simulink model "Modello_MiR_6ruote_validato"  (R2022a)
settings: Solver=VariableStepAuto  StartTime=0.0  StopTime=time_s(end,1)  RelTol=1e-3
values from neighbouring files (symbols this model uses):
  a = 0.250    (= 0.25)    [Modello_MiR_6ruote_validato_script.m]    (also in Modello_MiR_2ruote_script.m; Modello_MiR_6ruote_script.m; Modello_MiR_UR_script.m)
  a1 = 0.18265    [Modello_MiR_6ruote_validato_script.m]    (also in Modello_MiR_2ruote_script.m = deg2rad(5); Modello_MiR_6ruote_script.m = deg2rad(5); Modello_MiR_UR_script.m; UR_DHtable_e.m = 0)
  a2 = 0.40857    [Modello_MiR_6ruote_validato_script.m]    (also in Modello_MiR_2ruote_script.m = deg2rad(25); Modello_MiR_6ruote_script.m = deg2rad(25); Modello_MiR_UR_script.m; UR_DHtable_e.m = 612)
  Att_C1 = 0.01    [Modello_MiR_6ruote_validato_script.m]    (also in Modello_MiR_UR_script.m)
  Att_C2 = 0.01    [Modello_MiR_6ruote_validato_script.m]    (also in Modello_MiR_UR_script.m)
  Att_C5 = 0.01    [Modello_MiR_6ruote_validato_script.m]    (also in Modello_MiR_UR_script.m)
  Att_C6 = 0.01    [Modello_MiR_6ruote_validato_script.m]    (also in Modello_MiR_UR_script.m)
  b = 0.1875    [Modello_MiR_6ruote_validato_script.m]    (also in Modello_MiR_2ruote_script.m; Modello_MiR_6ruote_script.m; Modello_MiR_UR_script.m)
  b_caster = 0.07    [Modello_MiR_6ruote_validato_script.m]    (also in Modello_MiR_2ruote_script.m; Modello_MiR_6ruote_script.m; Modello_MiR_UR_script.m)
  bd = 0.205    [Modello_MiR_6ruote_validato_script.m]    (also in Modello_MiR_2ruote_script.m; Modello_MiR_6ruote_script.m; Modello_MiR_UR_script.m)
  F23fun = @(u) (mv*9.801/4)-(mv*h*u(5)+(mv*9.801/4)*(2*a-b_caster*(cos(u(1))+cos(u(2)))))/(4*a-b_caster*(cos(u(1))+cos(u(2)))+b_caster*(cos(u(3))+cos(u(4))))    [Modello_MiR_6ruote_validato_script.m]    (also in Modello_MiR_6ruote_script.m = @(u) (mv*9.801/4)-u(7))
  F43fun = @(u) (1/(2*bd))*(mv*u(6)*h+((mv*h*u(5)+(mv*9.801/4)*(2*a-b_caster*(cos(u(1))+cos(u(2)))))/(4*a-b_caster*(cos(u(1))+cos(u(2)))+b_caster*(cos(u(3))+cos(u(4)))))*(2*bd-b_caster*(sin(u(3))+sin(u(4))))+((mv*9.801/4)-(mv*h*u(5)+(mv*9.801/4)*(2*a-b_caster*(cos(u(1))+cos(u(2)))))/(4*a-b_caster*(cos(u(1))+cos(u(2)))+b_caster*(cos(u(3))+cos(u(4)))))*(2*bd-b_caster*(sin(u(1))+sin(u(2)))))    [Modello_MiR_6ruote_validato_script.m]    (also in Modello_MiR_6ruote_script.m = @(u) (1/(2*bd))*(mv*u(6)*h+u(7)*(2*bd-b_caster*(sin(u(3))+si)
  F63fun = @(u) (mv*h*u(5)+(mv*9.801/4)*(2*a-b_caster*(cos(u(1))+cos(u(2)))))/(4*a-b_caster*(cos(u(1))+cos(u(2)))+b_caster*(cos(u(3))+cos(u(4))))    [Modello_MiR_6ruote_validato_script.m]    (also in Modello_MiR_6ruote_script.m)
  f_c = 0.29564    [Modello_MiR_6ruote_validato_script.m]    (also in Modello_MiR_UR_script.m)
  f_d3 = 0.35846    [Modello_MiR_6ruote_validato_script.m]    (also in Modello_MiR_UR_script.m)
  f_d4 = 0.2333    [Modello_MiR_6ruote_validato_script.m]    (also in Modello_MiR_UR_script.m)
  fa_c = 0.27474    [Modello_MiR_6ruote_validato_script.m]    (also in Modello_MiR_UR_script.m)
  fa_d3 = 0.3694    [Modello_MiR_6ruote_validato_script.m]    (also in Modello_MiR_UR_script.m)
  fa_d4 = 0.28065    [Modello_MiR_6ruote_validato_script.m]    (also in Modello_MiR_UR_script.m)
  fm_fun = @(u) (u <= -am2 || u >= am2) * 0 + (u > -am2 && u <= -am1) * (- u* Mza/(am2 -am1) - Mza* am2/(am2 -am1)) +           + (u > -am1 && u <= am1) * (Mza * u / am1) + (u > am1 && u < am2) * (Mza * u /(am1 -am2) - Mza * am2 /(am1 - am2))    [Modello_MiR_6ruote_validato_script.m]    (also in Modello_MiR_6ruote_script.m = @(u) (u <= -am2 | u >= am2)*0 + (u > -am2 && u <= -am1)*(- u; Modello_MiR_UR_script.m)
  Icw_1 = 1/2 * mcw * rc^2    (= 0.002004225735)    [Modello_MiR_6ruote_validato_script.m]    (also in Modello_MiR_2ruote_script.m; Modello_MiR_6ruote_script.m; Modello_MiR_UR_script.m)
  Icw_2 = 1/12 * mcw * ec^2 + 1/4 * mcw * rc^2    (= 0.00104098243873)    [Modello_MiR_6ruote_validato_script.m]    (also in Modello_MiR_2ruote_script.m; Modello_MiR_6ruote_script.m; Modello_MiR_UR_script.m)
  Idw_1 = 1/2 * mdw * rd^2    (= 0.00551836278784)    [Modello_MiR_6ruote_validato_script.m]    (also in Modello_MiR_2ruote_script.m; Transfer_Function_Gol_Gcl.m = Inertia_vect(jj,1); Modello_MiR_6ruote_script.m; Modello_MiR_UR_script.m)
  iMax = 20.7*1.1    (= 22.77)    [Modello_MiR_6ruote_validato_script.m]    (also in Modello_MiR_2ruote_script.m; Modello_MiR_6ruote_script.m; Modello_MiR_UR_script.m)
  Iv = mv * (l^2 + w^2)  / 12    (= 8.95033333333)    [Modello_MiR_6ruote_validato_script.m]    (also in Modello_MiR_2ruote_script.m = 6.75343333333; Modello_MiR_6ruote_script.m = 6.75343333333; Modello_MiR_UR_script.m = 6.75343333333)
  Kc = 0.15    [Modello_MiR_6ruote_validato_script.m]    (also in Modello_MiR_2ruote_script.m; Modello_MiR_6ruote_script.m; Modello_MiR_UR_script.m)
  Ki_i = 1    [Modello_MiR_6ruote_validato_script.m]    (also in Modello_MiR_2ruote_script.m; Modello_MiR_6ruote_script.m; Modello_MiR_UR_script.m)
  Ki_v = 1    [Modello_MiR_6ruote_validato_script.m]    (also in Modello_MiR_2ruote_script.m; Modello_MiR_6ruote_script.m; Modello_MiR_UR_script.m)
  kk = 0.00005    (= 5e-05)    [Modello_MiR_6ruote_validato_script.m]    (also in Modello_MiR_2ruote_script.m; Modello_MiR_6ruote_script.m; Modello_MiR_UR_script.m)
  Kp_i = 5    [Modello_MiR_6ruote_validato_script.m]    (also in Modello_MiR_2ruote_script.m; Modello_MiR_6ruote_script.m; Modello_MiR_UR_script.m)
  Kp_v = 5    [Modello_MiR_6ruote_validato_script.m]    (also in Modello_MiR_2ruote_script.m; Modello_MiR_6ruote_script.m; Modello_MiR_UR_script.m)
  kv = 1.5e-6    (= 1.5e-06)    [Modello_MiR_6ruote_validato_script.m]    (also in Modello_MiR_2ruote_script.m; Modello_MiR_6ruote_script.m; Modello_MiR_UR_script.m)
  L = R * tauE    (= 0.00181134822805)    [Modello_MiR_6ruote_validato_script.m]    (also in Modello_MiR_2ruote_script.m; Modello_MiR_6ruote_script.m; Modello_MiR_UR_script.m)
  mcw = rc^2 * pi * ec * rhopoliu + 1    (= 1.02616357632)    [Modello_MiR_6ruote_validato_script.m]    (also in Modello_MiR_2ruote_script.m; Modello_MiR_6ruote_script.m; Modello_MiR_UR_script.m)
  mv = 110    [Modello_MiR_6ruote_validato_script.m]    (also in Modello_MiR_2ruote_script.m = 83; Modello_MiR_6ruote_script.m = 83; Modello_MiR_UR_script.m = 83)
  Phi1_start = psi_mir(1,1)    [Modello_MiR_6ruote_validato_script.m]    (also in Modello_MiR_UR_script.m)
  Phi2_start = psi_mir(1,1)    [Modello_MiR_6ruote_validato_script.m]    (also in Modello_MiR_UR_script.m)
  Phi5_start = psi_mir(1,1)    [Modello_MiR_6ruote_validato_script.m]    (also in Modello_MiR_UR_script.m)
  Phi6_start = psi_mir(1,1)    [Modello_MiR_6ruote_validato_script.m]    (also in Modello_MiR_UR_script.m)
  Psi_start = psi_mir(1,1)    [Modello_MiR_6ruote_validato_script.m]    (also in Modello_MiR_6ruote_script.m = 1.57079632679; Modello_MiR_UR_script.m)
  R = velMax * TorqueMax / (iMax)^2    (= 1.81134822805)    [Modello_MiR_6ruote_validato_script.m]    (also in Modello_MiR_2ruote_script.m; Modello_MiR_6ruote_script.m; Modello_MiR_UR_script.m)
  rap_rid = 10.167    [Modello_MiR_6ruote_validato_script.m]    (also in Modello_MiR_2ruote_script.m; Modello_MiR_6ruote_script.m; Modello_MiR_UR_script.m)
  rc = 0.125/2    (= 0.0625)    [Modello_MiR_6ruote_validato_script.m]    (also in Modello_MiR_2ruote_script.m; Modello_MiR_6ruote_script.m; Modello_MiR_UR_script.m)
  rd = 0.1    [Modello_MiR_6ruote_validato_script.m]    (also in Modello_MiR_2ruote_script.m; Modello_MiR_6ruote_script.m; Modello_MiR_UR_script.m)
  s1 = 0.18987    [Modello_MiR_6ruote_validato_script.m]    (also in Modello_MiR_2ruote_script.m = 0.2; Modello_MiR_6ruote_script.m = 0.2; Modello_MiR_UR_script.m)
  s2 = 0.99533    [Modello_MiR_6ruote_validato_script.m]    (also in Modello_MiR_2ruote_script.m = 0.8; Modello_MiR_6ruote_script.m = 0.8; Modello_MiR_UR_script.m)
  Sx = spline(x ,fl_fun(x),zx)    [Modello_MiR_6ruote_script.m]
  Sy = spline(x ,ft_fun(x),zy)    [Modello_MiR_6ruote_script.m]
  VaMax = Kc * velMax    (= 41.2443991527)    [Modello_MiR_6ruote_validato_script.m]    (also in Modello_MiR_2ruote_script.m; Modello_MiR_6ruote_script.m; Modello_MiR_UR_script.m)
  X_start = traj(1,1)    [Modello_MiR_6ruote_validato_script.m]    (also in Modello_MiR_2ruote_script.m = input('Inserire coordinata x iniziale'); Modello_MiR_6ruote_script.m = input('Inserire coordinata x iniziale'); Modello_MiR_UR_script.m)
  Y_start = traj(1,2)    [Modello_MiR_6ruote_validato_script.m]    (also in Modello_MiR_2ruote_script.m = input('Inserire coordinata y iniziale'); Modello_MiR_6ruote_script.m = input('Inserire coordinata y iniziale'); Modello_MiR_UR_script.m)
undefined symbols (not defined in the file or in its folder): z
libraries: slpidlib x4
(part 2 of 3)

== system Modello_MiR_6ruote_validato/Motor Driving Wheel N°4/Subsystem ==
  Thetad_SET : Inport
  Thetad_FB : Inport  Port=2
  iFB : Inport  Port=3
  " " : slpidlib/PID Controller  Controller=PID  Form=Parallel  TimeDomain=Continuous-time  UseExternalTs=off  SampleTime=-1  IntegratorMethod=Forward Euler  FilterMethod=Forward Euler  ControllerParametersSource=internal  P=Kp_v  I=Ki_v  UseKiTs=off  D=0  N=1  UseFilter=on  TunerSelectOption=Transfer Function Based (PID Tuner App)  InitialConditionSource=internal  InitialConditionForIntegrator=0  InitialConditionForFilter=0  DifferentiatorICPrevScaledInput=0  ExternalReset=none  TrackingMode=off  Kt=1  LimitOutput=on  SatLimitsSource=internal  UpperSaturationLimit=iMax  LowerSaturationLimit=-iMax  LinearizeAsGain=on  AntiWindupMode=back-calculation  Kb=1  POutMin=[]  POutMax=[]  IOutMin=[]  IOutMax=[]  DOutMin=[]  DOutMax=[]  NOutMin=[]  NOutMax=[]  SumOutMin=[]  SumOutMax=[]  SaturationOutMin=[]  SaturationOutMax=[]  PParamMin=0  PParamMax=[]  IParamMin=0  IParamMax=[]  DParamMin=0  DParamMax=[]  NParamMin=[]  NParamMax=[]  KbParamMin=[]  KbParamMax=[]  KtParamMin=[]  KtParamMax=[]  KbOutMin=[]  KbOutMax=[]  KtOutMin=[]  KtOutMax=[]  IntegratorOutMin=[]  IntegratorOutMax=[]  FilterOutMin=[]  FilterOutMax=[]  SumI1OutMin=[]  SumI1OutMax=[]  SumI2OutMin=[]  SumI2OutMax=[]  SumI3OutMin=[]  SumI3OutMax=[]  SumI4OutMin=[]  SumI4OutMax=[]  SumDOutMin=[]  SumDOutMax=[]  DifferentiatorOutMin=[]  DifferentiatorOutMax=[]  FilterDiffOutCoefMin=[]  FilterDiffOutCoefMax=[]  ReciprocalOutMin=[]  ReciprocalOutMax=[]  SumDenOutMin=[]  SumDenOutMax=[]  SumNumOutMin=[]  SumNumOutMax=[]  DivideOutMin=[]  DivideOutMax=[]  UdiffTsProdOutMin=[]  UdiffTsProdOutMax=[]  NTsProdOutMin=[]  NTsProdOutMax=[]  UintegralTsProdOutMin=[]  UintegralTsProdOutMax=[]  UngainTsProdOutMin=[]  UngainTsProdOutMax=[]  IntegratorContinuousStateAttributes=''  IntegratorStateMustResolveToSignalObject=off  IntegratorRTWStateStorageClass=Auto  FilterContinuousStateAttributes=''  FilterStateMustResolveToSignalObject=off  FilterRTWStateStorageClass=Auto  ParallelPVariant=InternalParameters  IdealPVariant=Disabled  IVariant=InternalParameters  DVariant=InternalParameters  IntegratorVariant=Continuous  SatVariant=Enabled  AWVariant=BackCalculation  PCopyVariant=Disabled  TRVariant=Disabled  FdbkBlocksVariant=Forward  IdealPFdbkVariant=Disabled  SatFdbkVariant=Disabled  DerivativeFilterVariant=ContFilter  NVariant=InternalParameters  NCopyVariant=Disabled  FilterICVariant=InternalICsFilter  IntegratorICVariant=InternalICs  ExternalResetVariant=Disabled  TRSumVariant=Passthrough  SumFdbkVariant=Disabled  SumVariant=Sum_PID  TsampFilterVariant=InternalTs  TsampNgainVariant=Passthrough  TsampIntegralVariant=Passthrough  ExternalSaturationOutDataTypeStr=Inherit: Same as second input  aMode=0
  PID Controller1 : slpidlib/PID Controller  Controller=PID  Form=Parallel  TimeDomain=Continuous-time  UseExternalTs=off  SampleTime=-1  IntegratorMethod=Forward Euler  FilterMethod=Forward Euler  ControllerParametersSource=internal  P=Kp_i  I=Ki_i  UseKiTs=off  D=0  N=100  UseFilter=on  TunerSelectOption=Transfer Function Based (PID Tuner App)  InitialConditionSource=internal  InitialConditionForIntegrator=0  InitialConditionForFilter=0  DifferentiatorICPrevScaledInput=0  ExternalReset=none  TrackingMode=off  Kt=1  LimitOutput=on  SatLimitsSource=internal  UpperSaturationLimit=VaMax  LowerSaturationLimit=-VaMax  LinearizeAsGain=on  AntiWindupMode=back-calculation  Kb=1  POutMin=[]  POutMax=[]  IOutMin=[]  IOutMax=[]  DOutMin=[]  DOutMax=[]  NOutMin=[]  NOutMax=[]  SumOutMin=[]  SumOutMax=[]  SaturationOutMin=[]  SaturationOutMax=[]  PParamMin=[]  PParamMax=[]  IParamMin=[]  IParamMax=[]  DParamMin=[]  DParamMax=[]  NParamMin=[]  NParamMax=[]  KbParamMin=[]  KbParamMax=[]  KtParamMin=[]  KtParamMax=[]  KbOutMin=[]  KbOutMax=[]  KtOutMin=[]  KtOutMax=[]  IntegratorOutMin=[]  IntegratorOutMax=[]  FilterOutMin=[]  FilterOutMax=[]  SumI1OutMin=[]  SumI1OutMax=[]  SumI2OutMin=[]  SumI2OutMax=[]  SumI3OutMin=[]  SumI3OutMax=[]  SumI4OutMin=[]  SumI4OutMax=[]  SumDOutMin=[]  SumDOutMax=[]  DifferentiatorOutMin=[]  DifferentiatorOutMax=[]  FilterDiffOutCoefMin=[]  FilterDiffOutCoefMax=[]  ReciprocalOutMin=[]  ReciprocalOutMax=[]  SumDenOutMin=[]  SumDenOutMax=[]  SumNumOutMin=[]  SumNumOutMax=[]  DivideOutMin=[]  DivideOutMax=[]  UdiffTsProdOutMin=[]  UdiffTsProdOutMax=[]  NTsProdOutMin=[]  NTsProdOutMax=[]  UintegralTsProdOutMin=[]  UintegralTsProdOutMax=[]  UngainTsProdOutMin=[]  UngainTsProdOutMax=[]  IntegratorContinuousStateAttributes=''  IntegratorStateMustResolveToSignalObject=off  IntegratorRTWStateStorageClass=Auto  FilterContinuousStateAttributes=''  FilterStateMustResolveToSignalObject=off  FilterRTWStateStorageClass=Auto  ParallelPVariant=InternalParameters  IdealPVariant=Disabled  IVariant=InternalParameters  DVariant=InternalParameters  IntegratorVariant=Continuous  SatVariant=Enabled  AWVariant=BackCalculation  PCopyVariant=Disabled  TRVariant=Disabled  FdbkBlocksVariant=Forward  IdealPFdbkVariant=Disabled  SatFdbkVariant=Disabled  DerivativeFilterVariant=ContFilter  NVariant=InternalParameters  NCopyVariant=Disabled  FilterICVariant=InternalICsFilter  IntegratorICVariant=InternalICs  ExternalResetVariant=Disabled  TRSumVariant=Passthrough  SumFdbkVariant=Disabled  SumVariant=Sum_PID  TsampFilterVariant=InternalTs  TsampNgainVariant=Passthrough  TsampIntegralVariant=Passthrough  ExternalSaturationOutDataTypeStr=Inherit: Same as second input  aMode=0
  Scope : Scope  NumInputPorts=2
  Sum1 : Sum  Inputs=|+-
  Sum2 : Sum  Inputs=|+-
  VaRif : Outport  VectorParamsAs1DForOutWhenUnconnected=off
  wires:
  Thetad_FB/1 -> Scope/2, Sum1/2
  " "/1 -> Sum2/1
  PID Controller1/1 -> VaRif/1
  iFB/1 -> Sum2/2
  Thetad_SET/1 -> Scope/1, Sum1/1
  Sum1/1 -> " "/1
  Sum2/1 -> PID Controller1/1

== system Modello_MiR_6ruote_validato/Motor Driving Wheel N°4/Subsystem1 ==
  VaRif : Inport
  Thetad_FB : Inport  Port=2
  Add : Sum  Inputs=+--
  Gain : Gain  Gain=rap_rid
  Gain1 : Gain  Gain=1/L
  Gain2 : Gain  Gain=Kc
  Gain3 : Gain  Gain=R
  Gain4 : Gain  Gain=Kc
  Integrator : Integrator
  Scope : Scope
  Scope1 : Scope
  Torque Cm : Outport  VectorParamsAs1DForOutWhenUnconnected=off
  iFB : Outport  Port=2  VectorParamsAs1DForOutWhenUnconnected=off
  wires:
  VaRif/1 -> Add/1
  Add/1 -> Gain1/1
  Gain1/1 -> Integrator/1
  Integrator/1 -> Gain4/1, Gain3/1, iFB/1
  Gain3/1 -> Add/3
  Thetad_FB/1 -> Gain2/1, Scope/1
  Gain2/1 -> Add/2
  Gain4/1 -> Gain/1
  Gain/1 -> Scope1/1, Torque Cm/1

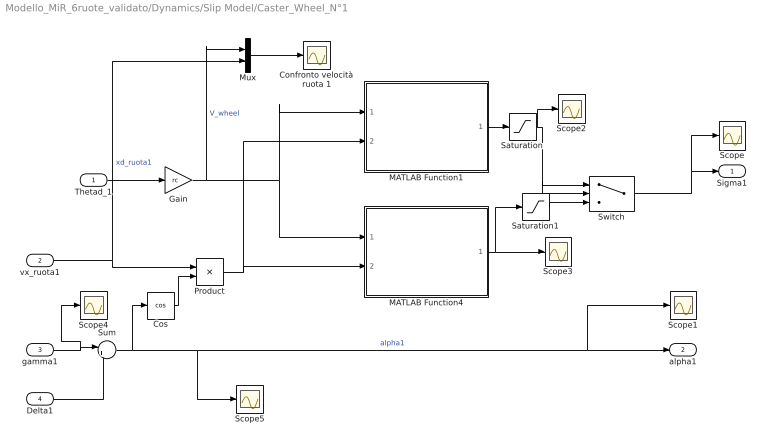
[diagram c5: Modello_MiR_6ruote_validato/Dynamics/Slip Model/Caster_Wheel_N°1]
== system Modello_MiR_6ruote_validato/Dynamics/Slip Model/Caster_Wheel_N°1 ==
  Thetad_1 : Inport
  vx_ruota1 : Inport  Port=2
  gamma1 : Inport  Port=3
  Delta1 : Inport  Port=4
  Confronto velocità ruota 1 : Scope
  Cos : Trigonometry  Operator=cos
  Gain : Gain  Gain=rc
  MATLAB Function1 : MATLAB Function  TreatAsAtomicUnit=on
  MATLAB Function4 : MATLAB Function  TreatAsAtomicUnit=on
  Mux : Mux  Inputs=2
  Product : Product
  Saturation : Saturate  UpperLimit=1  LowerLimit=-1
  Saturation1 : Saturate  UpperLimit=1  LowerLimit=-1
  Scope{,1..5} (6 alike) : Scope
  Sum : Sum  Inputs=|+-
  Switch : Switch
  Sigma1 : Outport
  alpha1 : Outport  Port=2
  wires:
  Thetad_1/1 -> Gain/1
  Gain/1 -> Mux/1, MATLAB Function4/1(v_wheel), MATLAB Function1/1(v_wheel)  "V_wheel"
  Switch/1 -> Scope/1, Sigma1/1
  MATLAB Function1/1(Fc_pos_out) -> Saturation/1
  MATLAB Function4/1(Fc_neg_out) -> Saturation1/1, Scope3/1
  vx_ruota1/1 -> Product/1, Mux/2  "xd_ruota1"
  Delta1/1 -> Sum/2
  Sum/1 -> Cos/1, Scope1/1, alpha1/1, Scope5/1  "alpha1"
  Mux/1 -> Confronto velocità ruota 1/1
  Saturation/1 -> Scope2/1, Switch/1, Switch/2
  Saturation1/1 -> Switch/3
  gamma1/1 -> Scope4/1, Sum/1
  Product/1 -> MATLAB Function1/2(Vx_DL), MATLAB Function4/2(Vx_DL)
  Cos/1 -> Product/2

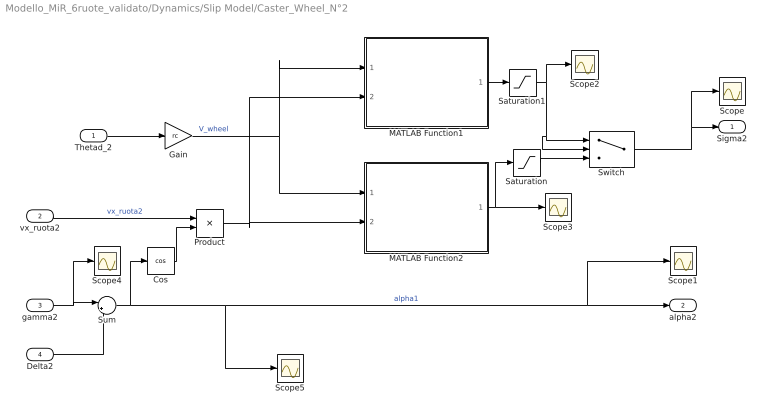
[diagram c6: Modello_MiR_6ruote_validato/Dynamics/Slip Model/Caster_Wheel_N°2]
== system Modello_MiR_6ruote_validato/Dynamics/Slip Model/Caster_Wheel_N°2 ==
  Thetad_2 : Inport
  vx_ruota2 : Inport  Port=2
  gamma2 : Inport  Port=3
  Delta2 : Inport  Port=4
  Cos : Trigonometry  Operator=cos
  Gain : Gain  Gain=rc
  MATLAB Function1 : MATLAB Function  TreatAsAtomicUnit=on
  MATLAB Function2 : MATLAB Function  TreatAsAtomicUnit=on
  Product : Product
  Saturation : Saturate  UpperLimit=1  LowerLimit=-1
  Saturation1 : Saturate  UpperLimit=1  LowerLimit=-1
  Scope{,1..5} (6 alike) : Scope
  Sum : Sum  Inputs=|+-
  Switch : Switch
  Sigma2 : Outport
  alpha2 : Outport  Port=2
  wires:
  Thetad_2/1 -> Gain/1
  gamma2/1 -> Scope4/1, Sum/1
  Gain/1 -> MATLAB Function2/1(v_wheel), MATLAB Function1/1(v_wheel)  "V_wheel"
  Switch/1 -> Scope/1, Sigma2/1
  MATLAB Function1/1(Fc_pos_out) -> Saturation1/1
  MATLAB Function2/1(Fc_neg_out) -> Saturation/1, Scope3/1
  Delta2/1 -> Sum/2
  Saturation1/1 -> Scope2/1, Switch/2, Switch/1
  Saturation/1 -> Switch/3
  Cos/1 -> Product/2
  Sum/1 -> Cos/1, Scope1/1, alpha2/1, Scope5/1  "alpha1"
  Product/1 -> MATLAB Function1/2(Vx_DL), MATLAB Function2/2(Vx_DL)
  vx_ruota2/1 -> Product/1  "vx_ruota2"

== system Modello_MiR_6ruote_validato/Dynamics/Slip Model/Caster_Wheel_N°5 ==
  Thetad_5 : Inport
  vx_ruota5 : Inport  Port=2
  gamma5 : Inport  Port=3
  Delta5 : Inport  Port=4
  Cos : Trigonometry  Operator=cos
  Gain : Gain  Gain=rc
  MATLAB Function1 : MATLAB Function  TreatAsAtomicUnit=on
  MATLAB Function4 : MATLAB Function  TreatAsAtomicUnit=on
  Product : Product
  Saturation : Saturate  UpperLimit=1  LowerLimit=-1
  Saturation1 : Saturate  UpperLimit=1  LowerLimit=-1
  Scope{,1..3} (4 alike) : Scope
  Sum : Sum  Inputs=|+-
  Switch : Switch
  Sigma5 : Outport
  alpha5 : Outport  Port=2
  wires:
  Thetad_5/1 -> Gain/1
  gamma5/1 -> Sum/1
  Gain/1 -> MATLAB Function4/1(v_wheel), MATLAB Function1/1(v_wheel)  "V_wheel"
  Switch/1 -> Scope/1, Sigma5/1
  MATLAB Function1/1(Fc_pos_out) -> Saturation/1
  MATLAB Function4/1(Fc_neg_out) -> Saturation1/1, Scope3/1
  Delta5/1 -> Sum/2
  Saturation/1 -> Scope2/1, Switch/1, Switch/2
  Saturation1/1 -> Switch/3
  Cos/1 -> Product/2
  Sum/1 -> Cos/1, Scope1/1, alpha5/1  "alpha1"
  Product/1 -> MATLAB Function1/2(Vx_DL), MATLAB Function4/2(Vx_DL)
  vx_ruota5/1 -> Product/1  "vx_ruota5"

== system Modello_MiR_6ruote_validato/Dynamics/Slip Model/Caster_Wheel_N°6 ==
  Thetad_6 : Inport
  vx_ruota6 : Inport  Port=2
  gamma6 : Inport  Port=3
  Delta6 : Inport  Port=4
  Cos : Trigonometry  Operator=cos
  Gain : Gain  Gain=rc
  MATLAB Function1 : MATLAB Function  TreatAsAtomicUnit=on
  MATLAB Function4 : MATLAB Function  TreatAsAtomicUnit=on
  Product : Product
  Saturation : Saturate  UpperLimit=1  LowerLimit=-1
  Saturation1 : Saturate  UpperLimit=1  LowerLimit=-1
  Scope{,1..3} (4 alike) : Scope
  Sum : Sum  Inputs=|+-
  Switch : Switch
  Sigma6 : Outport
  alpha6 : Outport  Port=2
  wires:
  Thetad_6/1 -> Gain/1
  gamma6/1 -> Sum/1
  Gain/1 -> MATLAB Function4/1(v_wheel), MATLAB Function1/1(v_wheel)  "V_wheel"
  Switch/1 -> Scope/1, Sigma6/1
  MATLAB Function1/1(Fc_pos_out) -> Saturation/1
  MATLAB Function4/1(Fc_neg_out) -> Saturation1/1, Scope3/1
  Delta6/1 -> Sum/2
  Saturation/1 -> Scope2/1, Switch/1, Switch/2
  Saturation1/1 -> Switch/3
  Cos/1 -> Product/2
  Sum/1 -> Cos/1, Scope1/1, alpha6/1  "alpha1"
  Product/1 -> MATLAB Function1/2(Vx_DL), MATLAB Function4/2(Vx_DL)
  vx_ruota6/1 -> Product/1  "xd_ruota6"

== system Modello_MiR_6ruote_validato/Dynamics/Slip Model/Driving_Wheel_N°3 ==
  Thetad_3 : Inport
  vx_ruota3 : Inport  Port=2
  gamma3 : Inport  Port=3
  Gain : Gain  Gain=rd
  MATLAB Function1 : MATLAB Function  TreatAsAtomicUnit=on
  MATLAB Function4 : MATLAB Function  TreatAsAtomicUnit=on
  Mux : Mux  Inputs=2
  Saturation : Saturate  UpperLimit=1  LowerLimit=-1
  Saturation1 : Saturate  UpperLimit=1  LowerLimit=-1
  Scope{,1..5} (6 alike) : Scope
  Switch : Switch
  Sigma3 : Outport
  alpha3 : Outport  Port=2
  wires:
  Thetad_3/1 -> Gain/1
  Gain/1 -> Mux/1, MATLAB Function4/1(v_wheel), MATLAB Function1/1(v_wheel)  "V_wheel"
  Switch/1 -> Scope/1, Sigma3/1
  MATLAB Function1/1(Fc_pos_out) -> Saturation1/1
  MATLAB Function4/1(Fc_neg_out) -> Saturation/1, Scope3/1
  vx_ruota3/1 -> MATLAB Function1/2(Vx_DL), MATLAB Function4/2(Vx_DL), Mux/2  "xd_ruota3"
  Saturation1/1 -> Scope2/1, Switch/1, Switch/2
  Saturation/1 -> Switch/3
  gamma3/1 -> Scope1/1, alpha3/1, Scope4/1
  Mux/1 -> Scope5/1

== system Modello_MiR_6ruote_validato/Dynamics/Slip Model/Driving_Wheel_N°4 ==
  Thetad_4 : Inport
  vx_ruota4 : Inport  Port=2
  gamma4 : Inport  Port=3
  Gain : Gain  Gain=rd
  MATLAB Function1 : MATLAB Function  TreatAsAtomicUnit=on
  MATLAB Function4 : MATLAB Function  TreatAsAtomicUnit=on
  Saturation : Saturate  UpperLimit=1  LowerLimit=-1
  Saturation1 : Saturate  UpperLimit=1  LowerLimit=-1
  Scope{,1..4} (5 alike) : Scope
  Switch : Switch
  Sigma4 : Outport
  alpha4 : Outport  Port=2
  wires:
  Thetad_4/1 -> Gain/1
  Gain/1 -> MATLAB Function4/1(v_wheel), MATLAB Function1/1(v_wheel)  "V_wheel"
  Switch/1 -> Scope/1, Sigma4/1
  MATLAB Function1/1(Fc_pos_out) -> Saturation1/1
  MATLAB Function4/1(Fc_neg_out) -> Saturation/1
  vx_ruota4/1 -> MATLAB Function4/2(Vx_DL), MATLAB Function1/2(Vx_DL)  "xd_ruota4"
  Saturation1/1 -> Scope2/1, Switch/1, Switch/2
  Saturation/1 -> Switch/3, Scope3/1
  gamma4/1 -> Scope1/1, alpha4/1, Scope4/1

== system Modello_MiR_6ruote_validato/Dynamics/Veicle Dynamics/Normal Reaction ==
  Delta1 : Inport
  Delta2 : Inport  Port=2
  Delta5 : Inport  Port=3
  Delta6 : Inport  Port=4
  a_tau : Inport  Port=5
  a_n : Inport  Port=6
  Interpreted MATLAB Function : MATLABFcn  MATLABFcn=F63fun(u)
  Interpreted MATLAB Function1 : MATLABFcn  MATLABFcn=F23fun(u)
  Interpreted MATLAB Function2 : MATLABFcn  MATLABFcn=F43fun(u)
  Interpreted MATLAB Function3 : MATLABFcn  MATLABFcn=mv*9.801-2*F63fun(u)-2*F23fun(u)-F43fun(u)
  Mux9 : Mux  Inputs=6
  Saturation{,1..3} (4 alike) : Saturate  UpperLimit=inf  LowerLimit=0
  F13 : Outport  PortDimensions=1
  F23 : Outport  Port=2  PortDimensions=1
  F33 : Outport  Port=3  PortDimensions=1
  F43 : Outport  Port=4  PortDimensions=1
  F53 : Outport  Port=5  PortDimensions=1
  F63 : Outport  Port=6  PortDimensions=1
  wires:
  Delta1/1 -> Mux9/1
  a_n/1 -> Mux9/6
  Delta6/1 -> Mux9/4
  Interpreted MATLAB Function3/1 -> Saturation3/1
  Mux9/1 -> Interpreted MATLAB Function3/1, Interpreted MATLAB Function2/1, Interpreted MATLAB Function1/1, Interpreted MATLAB Function/1
  Delta5/1 -> Mux9/3
  a_tau/1 -> Mux9/5
  Interpreted MATLAB Function1/1 -> Saturation1/1  "F23"
  Delta2/1 -> Mux9/2
  Interpreted MATLAB Function/1 -> Saturation/1  "F63"
  Interpreted MATLAB Function2/1 -> Saturation2/1
  Saturation/1 -> F63/1, F53/1
  Saturation1/1 -> F23/1, F13/1
  Saturation2/1 -> F43/1
  Saturation3/1 -> F33/1

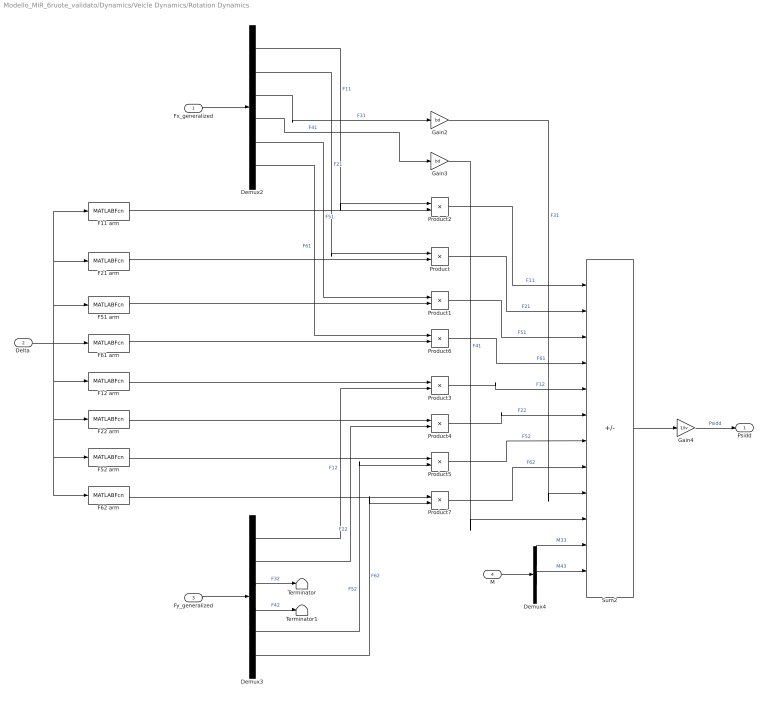
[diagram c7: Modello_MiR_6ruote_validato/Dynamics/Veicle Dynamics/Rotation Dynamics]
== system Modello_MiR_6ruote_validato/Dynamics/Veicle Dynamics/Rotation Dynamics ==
  Fx_generalized : Inport
  "Delta " : Inport  Port=2
  Fy_generalized : Inport  Port=3
  M : Inport  Port=4
  Demux2 : Demux  Outputs=6
  Demux3 : Demux  Outputs=6
  Demux4 : Demux  Outputs=2
  F11 arm : MATLABFcn  MATLABFcn=b-b_caster*sin(u(1))
  F12 arm : MATLABFcn  MATLABFcn=a-b_caster*cos(u(1))
  F21 arm : MATLABFcn  MATLABFcn=b+b_caster*sin(u(2))
  F22 arm : MATLABFcn  MATLABFcn=a-b_caster*cos(u(2))
  F51 arm : MATLABFcn  MATLABFcn=b-b_caster*sin(u(3))
  F52 arm : MATLABFcn  MATLABFcn=a+b_caster*cos(u(3))
  F61 arm : MATLABFcn  MATLABFcn=b+b_caster*sin(u(4))
  F62 arm : MATLABFcn  MATLABFcn=a+b_caster*cos(u(4))
  Gain2 : Gain  Gain=bd
  Gain3 : Gain  Gain=bd
  Gain4 : Gain  Gain=1/Iv
  Product{,1..7} (8 alike) : Product
  Sum2 : Sum  Inputs=-+-+++---+++
  Terminator : Terminator
  Terminator1 : Terminator
  Psidd : Outport  PortDimensions=1
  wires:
  Product2/1 -> Sum2/1  "F11"
  Demux3/2 -> Product4/2  "F22"
  Sum2/1 -> Gain4/1
  Demux3/3 -> Terminator/1  "F32"
  Product4/1 -> Sum2/6  "F22"
  Fx_generalized/1 -> Demux2/1
  Demux3/6 -> Product7/2  "F62"
  Demux2/2 -> Product/1  "F21"
  "Delta "/1 -> F51 arm/1, F21 arm/1, F11 arm/1, F62 arm/1, F52 arm/1, F22 arm/1, F12 arm/1, F61 arm/1
  Gain3/1 -> Sum2/10  "F41"
  Product7/1 -> Sum2/8  "F62"
  Gain2/1 -> Sum2/9  "F31"
  Product3/1 -> Sum2/5  "F12"
  Demux4/1 -> Sum2/11  "M33"
  Demux3/4 -> Terminator1/1  "F42"
  Demux4/2 -> Sum2/12  "M43"
  Demux2/1 -> Product2/1  "F11"
  Product/1 -> Sum2/2  "F21"
  Gain4/1 -> Psidd/1  "Psidd"
  Demux2/3 -> Gain2/1  "F31"
  Demux2/4 -> Gain3/1  "F41"
  F51 arm/1 -> Product1/2
  Demux3/5 -> Product5/2  "F52"
  F61 arm/1 -> Product6/2
  Demux2/5 -> Product1/1  "F51"
  Product5/1 -> Sum2/7  "F52"
  F21 arm/1 -> Product/2
  Demux3/1 -> Product3/2  "F12"
  Product1/1 -> Sum2/3  "F51"
  Demux2/6 -> Product6/1  "F61"
  F11 arm/1 -> Product2/2
  Product6/1 -> Sum2/4  "F61"
  Fy_generalized/1 -> Demux3/1
  F22 arm/1 -> Product4/1
  F52 arm/1 -> Product5/1
  F62 arm/1 -> Product7/1
  F12 arm/1 -> Product3/1
  M/1 -> Demux4/1

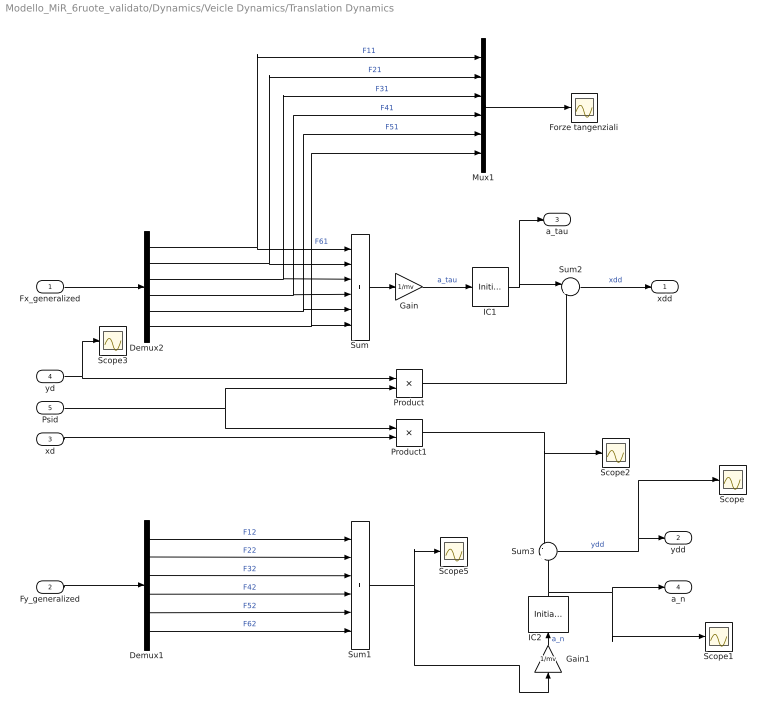
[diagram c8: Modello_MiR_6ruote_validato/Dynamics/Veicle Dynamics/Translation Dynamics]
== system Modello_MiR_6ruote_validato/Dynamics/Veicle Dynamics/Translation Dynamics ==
  Fx_generalized : Inport
  Fy_generalized : Inport  Port=2
  xd : Inport  Port=3
  yd : Inport  Port=4
  Psid : Inport  Port=5
  Demux1 : Demux  Outputs=6
  Demux2 : Demux  Outputs=6
  Forze tangenziali : Scope
  Gain : Gain  Gain=1/mv
  Gain1 : Gain  Gain=1/mv
  IC1 : InitialCondition  Value=0
  IC2 : InitialCondition  Value=0
  Mux1 : Mux  Inputs=6
  Product : Product
  Product1 : Product
  Scope{,1..3,5} (5 alike) : Scope
  Sum : Sum  Inputs=6
  Sum1 : Sum  Inputs=6
  Sum2 : Sum  Inputs=|++
  Sum3 : Sum  Inputs=-|+
  xdd : Outport  PortDimensions=1
  ydd : Outport  Port=2  PortDimensions=1
  a_tau : Outport  Port=3  PortDimensions=1
  a_n : Outport  Port=4  PortDimensions=1
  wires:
  Demux1/1 -> Sum1/1  "F12"
  Demux1/2 -> Sum1/2  "F22"
  Sum3/1 -> Scope/1, ydd/1  "ydd"
  Demux1/3 -> Sum1/3  "F32"
  Demux2/4 -> Mux1/4, Sum/4  "F41"
  Demux2/5 -> Mux1/5, Sum/5  "F51"
  Fx_generalized/1 -> Demux2/1
  Demux2/2 -> Sum/2, Mux1/2  "F21"
  Demux1/4 -> Sum1/4  "F42"
  Demux2/3 -> Sum/3, Mux1/3  "F31"
  Demux2/1 -> Sum/1, Mux1/1  "F11"
  Demux1/5 -> Sum1/5  "F52"
  Demux2/6 -> Mux1/6, Sum/6  "F61"
  Demux1/6 -> Sum1/6  "F62"
  Fy_generalized/1 -> Demux1/1
  Sum/1 -> Gain/1
  yd/1 -> Scope3/1, Product/1
  Psid/1 -> Product1/1, Product/2
  Gain/1 -> IC1/1  "a_tau"
  Product/1 -> Sum2/2
  xd/1 -> Product1/2
  Gain1/1 -> IC2/1  "a_n"
  Product1/1 -> Scope2/1, Sum3/1
  Sum1/1 -> Gain1/1, Scope5/1
  Mux1/1 -> Forze tangenziali/1
  IC1/1 -> Sum2/1, a_tau/1
  Sum2/1 -> xdd/1  "xdd"
  IC2/1 -> Sum3/2, Scope1/1, a_n/1

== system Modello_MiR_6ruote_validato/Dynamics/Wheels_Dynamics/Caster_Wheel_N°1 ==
  Sigma1 : Inport
  alpha1 : Inport  Port=2
  F13 : Inport  Port=3
  parametri_cw1 : Inport  Port=4
  Demux : Demux  Outputs=6
  Slip Forces/Torque : Subsystem
  Wheel Dynamics : Subsystem
  F1L : Outport
  F1T : Outport  Port=2
  Thetad_1 : Outport  Port=3
  Phid_1 : Outport  Port=4
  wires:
  Slip Forces/Torque/1(F1L) -> Wheel Dynamics/1(F1L), F1L/1  "F1L"
  alpha1/1 -> Slip Forces/Torque/2(Alpha1)
  Slip Forces/Torque/2(F1T) -> F1T/1
  Wheel Dynamics/2(Phid_1) -> Phid_1/1
  Sigma1/1 -> Slip Forces/Torque/1(Sigma1)
  Slip Forces/Torque/3(M13) -> Wheel Dynamics/2(M13)
  Wheel Dynamics/1(Thetad_1) -> Thetad_1/1
  F13/1 -> Wheel Dynamics/3(F13), Slip Forces/Torque/3(F13)
  Demux/1 -> Slip Forces/Torque/4(fc1)
  Demux/2 -> Slip Forces/Torque/5(fac1)
  Demux/3 -> Slip Forces/Torque/6(s1)
  Demux/6 -> Slip Forces/Torque/9(a2)
  Demux/5 -> Slip Forces/Torque/8(a1)
  Demux/4 -> Slip Forces/Torque/7(s2)
  parametri_cw1/1 -> Demux/1

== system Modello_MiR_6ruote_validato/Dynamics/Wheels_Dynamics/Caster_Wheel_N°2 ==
  Sigma2 : Inport
  alpha2 : Inport  Port=2
  F23 : Inport  Port=3
  parametri : Inport  Port=4
  Demux : Demux  Outputs=6
  Slip Forces/Torque : Subsystem
  Wheel Dynamics : Subsystem
  F2L : Outport
  F2T : Outport  Port=2
  Thetad_2 : Outport  Port=3
  Phid_2 : Outport  Port=4
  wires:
  Slip Forces/Torque/1(F2L) -> Wheel Dynamics/1(F2L), F2L/1
  alpha2/1 -> Slip Forces/Torque/2(Alpha2)
  Slip Forces/Torque/2(F2T) -> F2T/1
  Wheel Dynamics/2(Phid_2) -> Phid_2/1
  Sigma2/1 -> Slip Forces/Torque/1(Sigma2)
  Slip Forces/Torque/3(M23) -> Wheel Dynamics/2(M23)
  Wheel Dynamics/1(Thetad_2) -> Thetad_2/1
  F23/1 -> Slip Forces/Torque/3(F23), Wheel Dynamics/3(F23)
  Demux/1 -> Slip Forces/Torque/4(fc2)
  Demux/2 -> Slip Forces/Torque/5(fac2)
  Demux/3 -> Slip Forces/Torque/6(s1)
  Demux/4 -> Slip Forces/Torque/7(s2)
  Demux/5 -> Slip Forces/Torque/8(a1)
  Demux/6 -> Slip Forces/Torque/9(a2)
  parametri/1 -> Demux/1

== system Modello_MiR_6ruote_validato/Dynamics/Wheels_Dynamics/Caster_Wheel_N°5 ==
  Sigma5 : Inport
  alpha5 : Inport  Port=2
  F53 : Inport  Port=3
  parametri : Inport  Port=4
  Demux : Demux  Outputs=6
  Slip Forces/Torque : Subsystem
  Wheel Dynamics : Subsystem
  F5L : Outport
  F5T : Outport  Port=2
  Thetad_5 : Outport  Port=3
  Phid_5 : Outport  Port=4
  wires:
  alpha5/1 -> Slip Forces/Torque/2(Alpha5)
  Slip Forces/Torque/2(F5T) -> F5T/1
  Wheel Dynamics/2(Phid_5) -> Phid_5/1
  Sigma5/1 -> Slip Forces/Torque/1(Sigma5)
  Slip Forces/Torque/3(M53) -> Wheel Dynamics/2(M53)
  Wheel Dynamics/1(Thetad_5) -> Thetad_5/1
  F53/1 -> Slip Forces/Torque/3(F53), Wheel Dynamics/3(F53)
  Slip Forces/Torque/1(F5L) -> Wheel Dynamics/1(F5L), F5L/1
  Demux/6 -> Slip Forces/Torque/9(a2)
  Demux/4 -> Slip Forces/Torque/7(s2)
  Demux/1 -> Slip Forces/Torque/4(fc5)
  Demux/5 -> Slip Forces/Torque/8(a1)
  Demux/2 -> Slip Forces/Torque/5(fac5)
  Demux/3 -> Slip Forces/Torque/6(s1)
  parametri/1 -> Demux/1

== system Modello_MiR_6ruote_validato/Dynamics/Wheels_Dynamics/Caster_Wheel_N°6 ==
  Sigma6 : Inport
  alpha6 : Inport  Port=2
  F63 : Inport  Port=3
  parametri : Inport  Port=4
  Demux : Demux  Outputs=6
  Slip Forces/Torque : Subsystem
  Wheel Dynamics : Subsystem
  F6L : Outport
  F6T : Outport  Port=2
  Thetad_6 : Outport  Port=3
  Phid_6 : Outport  Port=4
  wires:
  Slip Forces/Torque/1(F6L) -> Wheel Dynamics/1(F6L), F6L/1
  alpha6/1 -> Slip Forces/Torque/2(Alpha6)
  Slip Forces/Torque/2(F6T) -> F6T/1
  Wheel Dynamics/2(Phid_6) -> Phid_6/1
  Sigma6/1 -> Slip Forces/Torque/1(Sigma6)
  Slip Forces/Torque/3(M63) -> Wheel Dynamics/2(M63)
  Wheel Dynamics/1(Thetad_6) -> Thetad_6/1
  F63/1 -> Slip Forces/Torque/3(F63), Wheel Dynamics/3(F63)
  Demux/6 -> Slip Forces/Torque/9(a2)
  Demux/4 -> Slip Forces/Torque/7(s2)
  Demux/1 -> Slip Forces/Torque/4(fc6)
  Demux/5 -> Slip Forces/Torque/8(a1)
  Demux/2 -> Slip Forces/Torque/5(fac6)
  Demux/3 -> Slip Forces/Torque/6(s1)
  parametri/1 -> Demux/1

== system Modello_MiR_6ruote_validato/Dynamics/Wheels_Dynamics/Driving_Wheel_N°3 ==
  Cm3 : Inport
  Sigma3 : Inport  Port=2
  alpha3 : Inport  Port=3
  F33 : Inport  Port=4
  parametri_dw3 : Inport  Port=5
  Demux : Demux  Outputs=6
  Scope : Scope
  Scope1 : Scope
  Scope2 : Scope
  Subsystem : Subsystem
  Wheel Dynamics : Subsystem
  F3L : Outport
  F3T : Outport  Port=2
  M33 : Outport  Port=3
  Thetad_3 : Outport  Port=4
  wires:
  Cm3/1 -> Wheel Dynamics/1(Cm3)
  Wheel Dynamics/1(Thetad_3) -> Thetad_3/1
  Sigma3/1 -> Subsystem/1(Sigma3)
  alpha3/1 -> Subsystem/2(alpha3)
  Subsystem/1(F3L) -> Scope/1, F3L/1, Wheel Dynamics/2(F3L)  "F3L"
  Subsystem/2(F3T) -> F3T/1, Scope2/1  "F3T"
  Subsystem/3(M33) -> Scope1/1, M33/1
  F33/1 -> Subsystem/3(F33), Wheel Dynamics/3(F33)
  Demux/6 -> Subsystem/9(a2)
  Demux/4 -> Subsystem/7(s2)
  Demux/1 -> Subsystem/4(f)
  Demux/5 -> Subsystem/8(a1)
  Demux/2 -> Subsystem/5(fa)
  Demux/3 -> Subsystem/6(s1)
  parametri_dw3/1 -> Demux/1

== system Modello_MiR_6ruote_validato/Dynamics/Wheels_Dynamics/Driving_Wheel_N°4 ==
  Cm4 : Inport
  Sigma4 : Inport  Port=2
  alpha4 : Inport  Port=3
  F43 : Inport  Port=4
  parametri_dw4 : Inport  Port=5
  Demux : Demux  Outputs=6
  Scope : Scope
  Scope1 : Scope
  Scope2 : Scope
  Subsystem : Subsystem
  Subsystem1 : Subsystem
  F4L : Outport
  F4T : Outport  Port=2
  M43 : Outport  Port=3
  Thetad_4 : Outport  Port=4
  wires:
  Cm4/1 -> Subsystem/1(Cm4)
  alpha4/1 -> Subsystem1/2(alpha4)
  Sigma4/1 -> Subsystem1/1(Sigma4)
  Subsystem1/1(F4L) -> Subsystem/2(F4L), Scope/1, F4L/1
  Subsystem1/2(F4T) -> Scope1/1, F4T/1
  Subsystem1/3(M43) -> Scope2/1, M43/1
  Subsystem/1(Thetad_4) -> Thetad_4/1
  F43/1 -> Subsystem1/3(F43), Subsystem/3(F43)
  Demux/6 -> Subsystem1/9(a2)
  Demux/4 -> Subsystem1/7(s2)
  Demux/1 -> Subsystem1/4(f)
  Demux/5 -> Subsystem1/8(a1)
  Demux/2 -> Subsystem1/5(fa)
  Demux/3 -> Subsystem1/6(s1)
  parametri_dw4/1 -> Demux/1

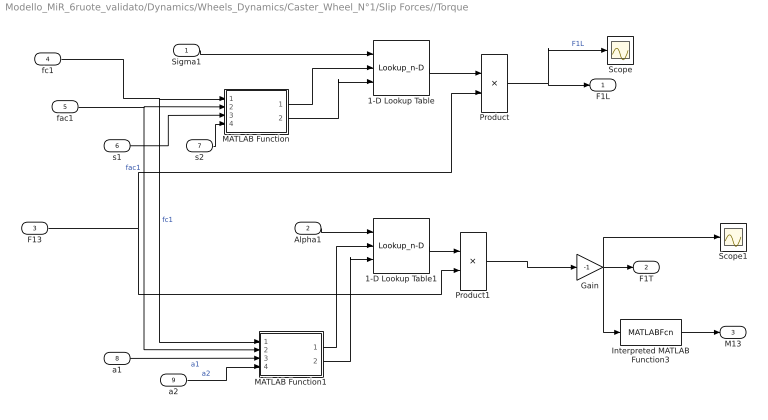
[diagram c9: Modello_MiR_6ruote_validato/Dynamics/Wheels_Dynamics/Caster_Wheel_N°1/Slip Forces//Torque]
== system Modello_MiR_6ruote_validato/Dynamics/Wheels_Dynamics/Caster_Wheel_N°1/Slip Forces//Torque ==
  Sigma1 : Inport
  Alpha1 : Inport  Port=2
  F13 : Inport  Port=3
  fc1 : Inport  Port=4
  fac1 : Inport  Port=5
  s1 : Inport  Port=6
  s2 : Inport  Port=7
  a1 : Inport  Port=8
  a2 : Inport  Port=9
  1-D Lookup Table : Lookup_n-D  NumberOfTableDimensions=1  BreakpointsForDimension1Source=Input port  BreakpointsForDimension1=z  TableSource=Input port  Table=Sx  InternalRulePriority=Speed  RndMeth=Simplest
  1-D Lookup Table1 : Lookup_n-D  NumberOfTableDimensions=1  BreakpointsForDimension1Source=Input port  BreakpointsForDimension1=z  TableSource=Input port  Table=Sy  InternalRulePriority=Speed  RndMeth=Simplest
  Gain : Gain  Gain=-1
  Interpreted MATLAB Function3 : MATLABFcn  MATLABFcn=u*b_caster
  MATLAB Function : MATLAB Function  TreatAsAtomicUnit=on
  MATLAB Function1 : MATLAB Function  TreatAsAtomicUnit=on
  Product : Product
  Product1 : Product
  Scope : Scope
  Scope1 : Scope
  F1L : Outport
  F1T : Outport  Port=2
  M13 : Outport  Port=3
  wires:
  F13/1 -> Product/2, Product1/2
  Product/1 -> F1L/1, Scope/1  "F1L"
  Product1/1 -> Gain/1
  Alpha1/1 -> 1-D Lookup Table1/1
  Interpreted MATLAB Function3/1 -> M13/1
  Gain/1 -> F1T/1, Scope1/1, Interpreted MATLAB Function3/1
  Sigma1/1 -> 1-D Lookup Table/1
  1-D Lookup Table/1 -> Product/1
  1-D Lookup Table1/1 -> Product1/1
  MATLAB Function/1(Sx) -> 1-D Lookup Table/2
  MATLAB Function/2(z) -> 1-D Lookup Table/3
  fc1/1 -> MATLAB Function1/1(f), MATLAB Function/1(f)  "fc1"
  fac1/1 -> MATLAB Function1/2(fa), MATLAB Function/2(fa)  "fac1"
  s1/1 -> MATLAB Function/3(s1)
  s2/1 -> MATLAB Function/4(s2)
  MATLAB Function1/1(Sy) -> 1-D Lookup Table1/2
  MATLAB Function1/2(z) -> 1-D Lookup Table1/3
  a1/1 -> MATLAB Function1/3(a1)  "a1"
  a2/1 -> MATLAB Function1/4(a2)  "a2"

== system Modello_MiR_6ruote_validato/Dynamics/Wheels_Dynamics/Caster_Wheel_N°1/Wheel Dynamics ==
  F1L : Inport
  M13 : Inport  Port=2
  F13 : Inport  Port=3
  Gain : Gain  Gain=-rc
  Gain1 : Gain  Gain=1/Icw_1
  Gain2 : Gain  Gain=1/(Icw_2+mcw*b_caster^2)
  Gain3 : Gain  Gain=Att_C1
  Integrator : Integrator
  Integrator1 : Integrator
  Interpreted MATLAB Function : MATLABFcn  MATLABFcn=u(2)*(kk*u(1)+kv*u(1)^2)  OutputDimensions=1
  Mux : Mux  Inputs=2
  Mux1 : Mux  Inputs=2
  Scope : Scope
  Scope1 : Scope
  Scope2 : Scope
  Sum : Sum  Inputs=+-
  Sum1 : Sum  Inputs=--
  Thetad_1 : Outport
  Phid_1 : Outport  Port=2  PortDimensions=1
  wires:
  Integrator/1 -> Mux/1, Thetad_1/1
  Sum/1 -> Scope/1, Gain1/1
  Gain1/1 -> Integrator/1
  F1L/1 -> Gain/1
  Gain/1 -> Sum/1
  Interpreted MATLAB Function/1 -> Sum/2
  M13/1 -> Sum1/1, Mux1/1  "M13"
  Sum1/1 -> Gain2/1
  Gain2/1 -> Integrator1/1
  Gain3/1 -> Mux1/2, Sum1/2  "Coppia_Attr"
  Mux/1 -> Interpreted MATLAB Function/1
  F13/1 -> Mux/2
  Mux1/1 -> Scope2/1
  Integrator1/1 -> Scope1/1, Phid_1/1, Gain3/1

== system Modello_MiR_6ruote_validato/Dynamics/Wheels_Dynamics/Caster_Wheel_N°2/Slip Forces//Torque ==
  Sigma2 : Inport
  Alpha2 : Inport  Port=2
  F23 : Inport  Port=3
  fc2 : Inport  Port=4
  fac2 : Inport  Port=5
  s1 : Inport  Port=6
  s2 : Inport  Port=7
  a1 : Inport  Port=8
  a2 : Inport  Port=9
  1-D Lookup Table : Lookup_n-D  NumberOfTableDimensions=1  BreakpointsForDimension1Source=Input port  BreakpointsForDimension1=z  TableSource=Input port  Table=Sx  InternalRulePriority=Speed  RndMeth=Simplest
  1-D Lookup Table1 : Lookup_n-D  NumberOfTableDimensions=1  BreakpointsForDimension1Source=Input port  BreakpointsForDimension1=z  TableSource=Input port  Table=Sy  InternalRulePriority=Speed  RndMeth=Simplest
  Gain : Gain  Gain=-1
  Interpreted MATLAB Function3 : MATLABFcn  MATLABFcn=b_caster*u
  MATLAB Function : MATLAB Function  TreatAsAtomicUnit=on
  MATLAB Function1 : MATLAB Function  TreatAsAtomicUnit=on
  Product : Product
  Product1 : Product
  Scope : Scope
  F2L : Outport
  F2T : Outport  Port=2
  M23 : Outport  Port=3
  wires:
  Product1/1 -> Gain/1
  Gain/1 -> Interpreted MATLAB Function3/1, F2T/1
  Sigma2/1 -> 1-D Lookup Table/1
  Alpha2/1 -> 1-D Lookup Table1/1
  Interpreted MATLAB Function3/1 -> M23/1
  Product/1 -> F2L/1, Scope/1  "F1L"
  F23/1 -> Product1/2, Product/2
  1-D Lookup Table1/1 -> Product1/1
  1-D Lookup Table/1 -> Product/1
  s1/1 -> MATLAB Function/3(s1)
  MATLAB Function/2(z) -> 1-D Lookup Table/3
  MATLAB Function/1(Sx) -> 1-D Lookup Table/2
  s2/1 -> MATLAB Function/4(s2)
  a1/1 -> MATLAB Function1/3(a1)
  MATLAB Function1/1(Sy) -> 1-D Lookup Table1/2
  MATLAB Function1/2(z) -> 1-D Lookup Table1/3
  fc2/1 -> MATLAB Function1/1(f), MATLAB Function/1(f)
  a2/1 -> MATLAB Function1/4(a2)
  fac2/1 -> MATLAB Function1/2(fa), MATLAB Function/2(fa)

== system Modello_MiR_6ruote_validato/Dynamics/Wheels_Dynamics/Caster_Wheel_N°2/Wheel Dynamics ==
  F2L : Inport
  M23 : Inport  Port=2
  F23 : Inport  Port=3
  Gain : Gain  Gain=-rc
  Gain1 : Gain  Gain=1/Icw_1
  Gain2 : Gain  Gain=1/(Icw_2+mcw*b_caster^2)
  Gain3 : Gain  Gain=Att_C2
  Integrator : Integrator
  Integrator1 : Integrator
  Interpreted MATLAB Function : MATLABFcn  MATLABFcn=u(2)*(kk*u(1)+kv*u(1)^2)  OutputDimensions=1
  Mux : Mux  Inputs=2
  Mux1 : Mux  Inputs=2
  Scope : Scope
  Scope2 : Scope
  Sum : Sum  Inputs=+-
  Sum1 : Sum  Inputs=--
  Thetad_2 : Outport
  Phid_2 : Outport  Port=2  PortDimensions=1
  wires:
  Integrator/1 -> Mux/1, Thetad_2/1
  Sum/1 -> Scope/1, Gain1/1
  Gain1/1 -> Integrator/1
  F2L/1 -> Gain/1
  Gain/1 -> Sum/1
  Interpreted MATLAB Function/1 -> Sum/2
  Sum1/1 -> Gain2/1
  Gain2/1 -> Integrator1/1
  Mux/1 -> Interpreted MATLAB Function/1
  F23/1 -> Mux/2
  Gain3/1 -> Mux1/2, Sum1/2  "Coppia_Attr"
  Mux1/1 -> Scope2/1
  M23/1 -> Sum1/1, Mux1/1  "M23"
  Integrator1/1 -> Gain3/1, Phid_2/1

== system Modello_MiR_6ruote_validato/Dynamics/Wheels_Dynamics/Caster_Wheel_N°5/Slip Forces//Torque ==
  Sigma5 : Inport
  Alpha5 : Inport  Port=2
  F53 : Inport  Port=3
  fc5 : Inport  Port=4
  fac5 : Inport  Port=5
  s1 : Inport  Port=6
  s2 : Inport  Port=7
  a1 : Inport  Port=8
  a2 : Inport  Port=9
  1-D Lookup Table : Lookup_n-D  NumberOfTableDimensions=1  BreakpointsForDimension1Source=Input port  BreakpointsForDimension1=z  TableSource=Input port  Table=Sx  InternalRulePriority=Speed  RndMeth=Simplest
  1-D Lookup Table1 : Lookup_n-D  NumberOfTableDimensions=1  BreakpointsForDimension1Source=Input port  BreakpointsForDimension1=z  TableSource=Input port  Table=Sy  InternalRulePriority=Speed  RndMeth=Simplest
  Gain : Gain  Gain=-1
  Interpreted MATLAB Function3 : MATLABFcn  MATLABFcn=b_caster*u
  MATLAB Function : MATLAB Function  TreatAsAtomicUnit=on
  MATLAB Function1 : MATLAB Function  TreatAsAtomicUnit=on
  Product : Product
  Product1 : Product
  F5L : Outport
  F5T : Outport  Port=2
  M53 : Outport  Port=3
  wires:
  Product1/1 -> Gain/1
  Gain/1 -> Interpreted MATLAB Function3/1, F5T/1
  Interpreted MATLAB Function3/1 -> M53/1
  Product/1 -> F5L/1  "F1L"
  1-D Lookup Table1/1 -> Product1/1
  1-D Lookup Table/1 -> Product/1
  Alpha5/1 -> 1-D Lookup Table1/1
  Sigma5/1 -> 1-D Lookup Table/1
  F53/1 -> Product1/2, Product/2
  s1/1 -> MATLAB Function/3(s1)
  MATLAB Function/2(z) -> 1-D Lookup Table/3
  MATLAB Function/1(Sx) -> 1-D Lookup Table/2
  s2/1 -> MATLAB Function/4(s2)
  a1/1 -> MATLAB Function1/3(a1)
  MATLAB Function1/1(Sy) -> 1-D Lookup Table1/2
  MATLAB Function1/2(z) -> 1-D Lookup Table1/3
  fc5/1 -> MATLAB Function/1(f), MATLAB Function1/1(f)
  a2/1 -> MATLAB Function1/4(a2)
  fac5/1 -> MATLAB Function1/2(fa), MATLAB Function/2(fa)

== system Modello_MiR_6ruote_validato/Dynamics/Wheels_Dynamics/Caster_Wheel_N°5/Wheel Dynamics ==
  F5L : Inport
  M53 : Inport  Port=2
  F53 : Inport  Port=3
  Gain : Gain  Gain=-rc
  Gain1 : Gain  Gain=1/Icw_1
  Gain2 : Gain  Gain=1/(Icw_2+mcw*b_caster^2)
  Gain3 : Gain  Gain=Att_C5
  Integrator : Integrator
  Integrator1 : Integrator
  Interpreted MATLAB Function : MATLABFcn  MATLABFcn=u(2)*(kk*u(1)+kv*u(1)^2)  OutputDimensions=1
  Mux : Mux  Inputs=2
  Mux1 : Mux  Inputs=2
  Scope : Scope
  Scope2 : Scope
  Sum : Sum  Inputs=+-
  Sum1 : Sum  Inputs=--
  Thetad_5 : Outport
  Phid_5 : Outport  Port=2  PortDimensions=1
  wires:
  Integrator/1 -> Mux/1, Thetad_5/1
  Sum/1 -> Scope/1, Gain1/1
  Gain1/1 -> Integrator/1
  F5L/1 -> Gain/1
  Gain/1 -> Sum/1
  Interpreted MATLAB Function/1 -> Sum/2
  Sum1/1 -> Gain2/1
  Gain2/1 -> Integrator1/1
  Mux/1 -> Interpreted MATLAB Function/1
  F53/1 -> Mux/2
  Gain3/1 -> Mux1/2, Sum1/2  "Coppia_Attr"
  Mux1/1 -> Scope2/1
  M53/1 -> Sum1/1, Mux1/1  "M53"
  Integrator1/1 -> Gain3/1, Phid_5/1

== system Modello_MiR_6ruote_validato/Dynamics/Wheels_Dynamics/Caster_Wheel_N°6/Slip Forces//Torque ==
  Sigma6 : Inport
  Alpha6 : Inport  Port=2
  F63 : Inport  Port=3
  fc6 : Inport  Port=4
  fac6 : Inport  Port=5
  s1 : Inport  Port=6
  s2 : Inport  Port=7
  a1 : Inport  Port=8
  a2 : Inport  Port=9
  1-D Lookup Table : Lookup_n-D  NumberOfTableDimensions=1  BreakpointsForDimension1Source=Input port  BreakpointsForDimension1=z  TableSource=Input port  Table=Sx  InternalRulePriority=Speed  RndMeth=Simplest
  1-D Lookup Table1 : Lookup_n-D  NumberOfTableDimensions=1  BreakpointsForDimension1Source=Input port  BreakpointsForDimension1=z  TableSource=Input port  Table=Sy  InternalRulePriority=Speed  RndMeth=Simplest
  Gain : Gain  Gain=-1
  Interpreted MATLAB Function1 : MATLABFcn  MATLABFcn=b_caster*u
  MATLAB Function : MATLAB Function  TreatAsAtomicUnit=on
  MATLAB Function1 : MATLAB Function  TreatAsAtomicUnit=on
  Product : Product
  Product1 : Product
  F6L : Outport
  F6T : Outport  Port=2
  M63 : Outport  Port=3
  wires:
  Product1/1 -> Gain/1
  Gain/1 -> Interpreted MATLAB Function1/1, F6T/1
  Interpreted MATLAB Function1/1 -> M63/1
  1-D Lookup Table1/1 -> Product1/1
  1-D Lookup Table/1 -> Product/1
  Product/1 -> F6L/1  "F1L"
  F63/1 -> Product/2, Product1/2
  Alpha6/1 -> 1-D Lookup Table1/1
  Sigma6/1 -> 1-D Lookup Table/1
  s1/1 -> MATLAB Function/3(s1)
  MATLAB Function/2(z) -> 1-D Lookup Table/3
  MATLAB Function/1(Sx) -> 1-D Lookup Table/2
  s2/1 -> MATLAB Function/4(s2)
  a1/1 -> MATLAB Function1/3(a1)
  MATLAB Function1/1(Sy) -> 1-D Lookup Table1/2
  MATLAB Function1/2(z) -> 1-D Lookup Table1/3
  fc6/1 -> MATLAB Function1/1(f), MATLAB Function/1(f)
  a2/1 -> MATLAB Function1/4(a2)
  fac6/1 -> MATLAB Function1/2(fa), MATLAB Function/2(fa)

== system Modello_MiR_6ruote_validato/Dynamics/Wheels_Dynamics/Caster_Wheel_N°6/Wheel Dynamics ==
  F6L : Inport
  M63 : Inport  Port=2
  F63 : Inport  Port=3
  Gain : Gain  Gain=-rc
  Gain1 : Gain  Gain=1/Icw_1
  Gain2 : Gain  Gain=1/(Icw_2+mcw*b_caster^2)
  Gain3 : Gain  Gain=Att_C6
  Integrator : Integrator
  Integrator1 : Integrator
  Interpreted MATLAB Function : MATLABFcn  MATLABFcn=u(2)*(kk*u(1)+kv*u(1)^2)  OutputDimensions=1
  Mux : Mux  Inputs=2
  Mux1 : Mux  Inputs=2
  Scope : Scope
  Scope2 : Scope
  Sum : Sum  Inputs=+-
  Sum1 : Sum  Inputs=--
  Thetad_6 : Outport
  Phid_6 : Outport  Port=2  PortDimensions=1
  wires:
  Integrator/1 -> Mux/1, Thetad_6/1
  Sum/1 -> Scope/1, Gain1/1
  Gain1/1 -> Integrator/1
  F6L/1 -> Gain/1
  Gain/1 -> Sum/1
  Interpreted MATLAB Function/1 -> Sum/2
  Sum1/1 -> Gain2/1
  Gain2/1 -> Integrator1/1
  Mux/1 -> Interpreted MATLAB Function/1
  F63/1 -> Mux/2
  Gain3/1 -> Mux1/2, Sum1/2  "Coppia_Attr"
  Mux1/1 -> Scope2/1
  M63/1 -> Sum1/1, Mux1/1  "M63"
  Integrator1/1 -> Gain3/1, Phid_6/1

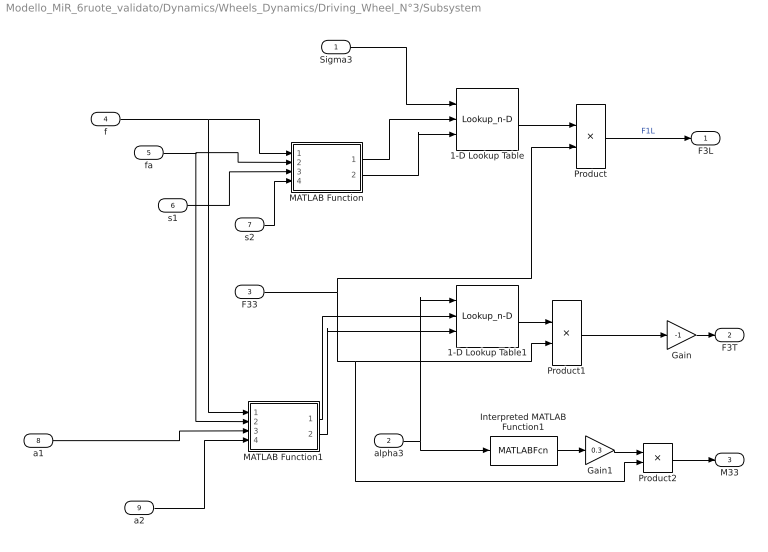
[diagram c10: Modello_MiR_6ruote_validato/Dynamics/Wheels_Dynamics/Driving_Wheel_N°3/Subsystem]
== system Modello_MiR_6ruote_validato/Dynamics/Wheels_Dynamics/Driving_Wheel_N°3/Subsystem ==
  Sigma3 : Inport
  alpha3 : Inport  Port=2
  F33 : Inport  Port=3
  f : Inport  Port=4
  fa : Inport  Port=5
  s1 : Inport  Port=6
  s2 : Inport  Port=7
  a1 : Inport  Port=8
  a2 : Inport  Port=9
  1-D Lookup Table : Lookup_n-D  NumberOfTableDimensions=1  BreakpointsForDimension1Source=Input port  BreakpointsForDimension1=z  TableSource=Input port  Table=Sx  InternalRulePriority=Speed  RndMeth=Simplest
  1-D Lookup Table1 : Lookup_n-D  NumberOfTableDimensions=1  BreakpointsForDimension1Source=Input port  BreakpointsForDimension1=z  TableSource=Input port  Table=Sy  InternalRulePriority=Speed  RndMeth=Simplest
  Gain : Gain  Gain=-1
  Gain1 : Gain  Gain=0.3
  Interpreted MATLAB Function1 : MATLABFcn  MATLABFcn=fm_fun(u)
  MATLAB Function : MATLAB Function  TreatAsAtomicUnit=on
  MATLAB Function1 : MATLAB Function  TreatAsAtomicUnit=on
  Product : Product
  Product1 : Product
  Product2 : Product
  F3L : Outport
  F3T : Outport  Port=2
  M33 : Outport  Port=3
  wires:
  Gain/1 -> F3T/1
  Interpreted MATLAB Function1/1 -> Gain1/1
  F33/1 -> Product2/2, Product1/2, Product/2
  alpha3/1 -> Interpreted MATLAB Function1/1, 1-D Lookup Table1/1
  Product1/1 -> Gain/1
  Product/1 -> F3L/1  "F1L"
  1-D Lookup Table1/1 -> Product1/1
  1-D Lookup Table/1 -> Product/1
  Sigma3/1 -> 1-D Lookup Table/1
  s1/1 -> MATLAB Function/3(s1)
  MATLAB Function/2(z) -> 1-D Lookup Table/3
  MATLAB Function/1(Sx) -> 1-D Lookup Table/2
  s2/1 -> MATLAB Function/4(s2)
  a1/1 -> MATLAB Function1/3(a1)
  MATLAB Function1/1(Sy) -> 1-D Lookup Table1/2
  MATLAB Function1/2(z) -> 1-D Lookup Table1/3
  f/1 -> MATLAB Function1/1(f), MATLAB Function/1(f)
  a2/1 -> MATLAB Function1/4(a2)
  fa/1 -> MATLAB Function1/2(fa), MATLAB Function/2(fa)
  Gain1/1 -> Product2/1
  Product2/1 -> M33/1

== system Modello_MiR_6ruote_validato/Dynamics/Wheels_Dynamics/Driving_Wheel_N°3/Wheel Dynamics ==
  Cm3 : Inport
  F3L : Inport  Port=2
  F33 : Inport  Port=3
  Gain : Gain  Gain=rd
  Gain1 : Gain  Gain=1/(Idw_1+2*10^(-3))
  Integrator : Integrator
  Interpreted MATLAB Function : MATLABFcn  MATLABFcn=u(2)*(kk*u(1)+kv*u(1)^2)  OutputDimensions=1
  Mux : Mux  Inputs=2
  Scope : Scope
  Sum : Sum  Inputs=+--
  Thetad_3 : Outport
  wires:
  Cm3/1 -> Sum/1
  Gain/1 -> Sum/2
  Interpreted MATLAB Function/1 -> Sum/3
  Integrator/1 -> Mux/1, Thetad_3/1
  Sum/1 -> Scope/1, Gain1/1
  Gain1/1 -> Integrator/1
  F3L/1 -> Gain/1
  Mux/1 -> Interpreted MATLAB Function/1
  F33/1 -> Mux/2

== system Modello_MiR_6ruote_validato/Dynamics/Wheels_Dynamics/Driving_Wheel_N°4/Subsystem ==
  Cm4 : Inport
  F4L : Inport  Port=2
  F43 : Inport  Port=3
  Gain : Gain  Gain=rd
  Gain1 : Gain  Gain=1/(Idw_1+2*10^(-3))
  Integrator : Integrator
  Interpreted MATLAB Function : MATLABFcn  MATLABFcn=u(2)*(kk*u(1)+kv*u(1)^2)  OutputDimensions=1
  Mux : Mux  Inputs=3
  Mux1 : Mux  Inputs=2
  Scope : Scope
  Sum : Sum  Inputs=+--
  Thetad_4 : Outport
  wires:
  Interpreted MATLAB Function/1 -> Mux/2, Sum/3  "Res_rot"
  Gain/1 -> Mux/3, Sum/2  "rd*Fc_R"
  Sum/1 -> Gain1/1
  Gain1/1 -> Integrator/1
  Integrator/1 -> Mux1/1, Thetad_4/1
  F4L/1 -> Gain/1
  Cm4/1 -> Mux/1, Sum/1  "Cm_R"
  Mux/1 -> Scope/1
  Mux1/1 -> Interpreted MATLAB Function/1
  F43/1 -> Mux1/2
